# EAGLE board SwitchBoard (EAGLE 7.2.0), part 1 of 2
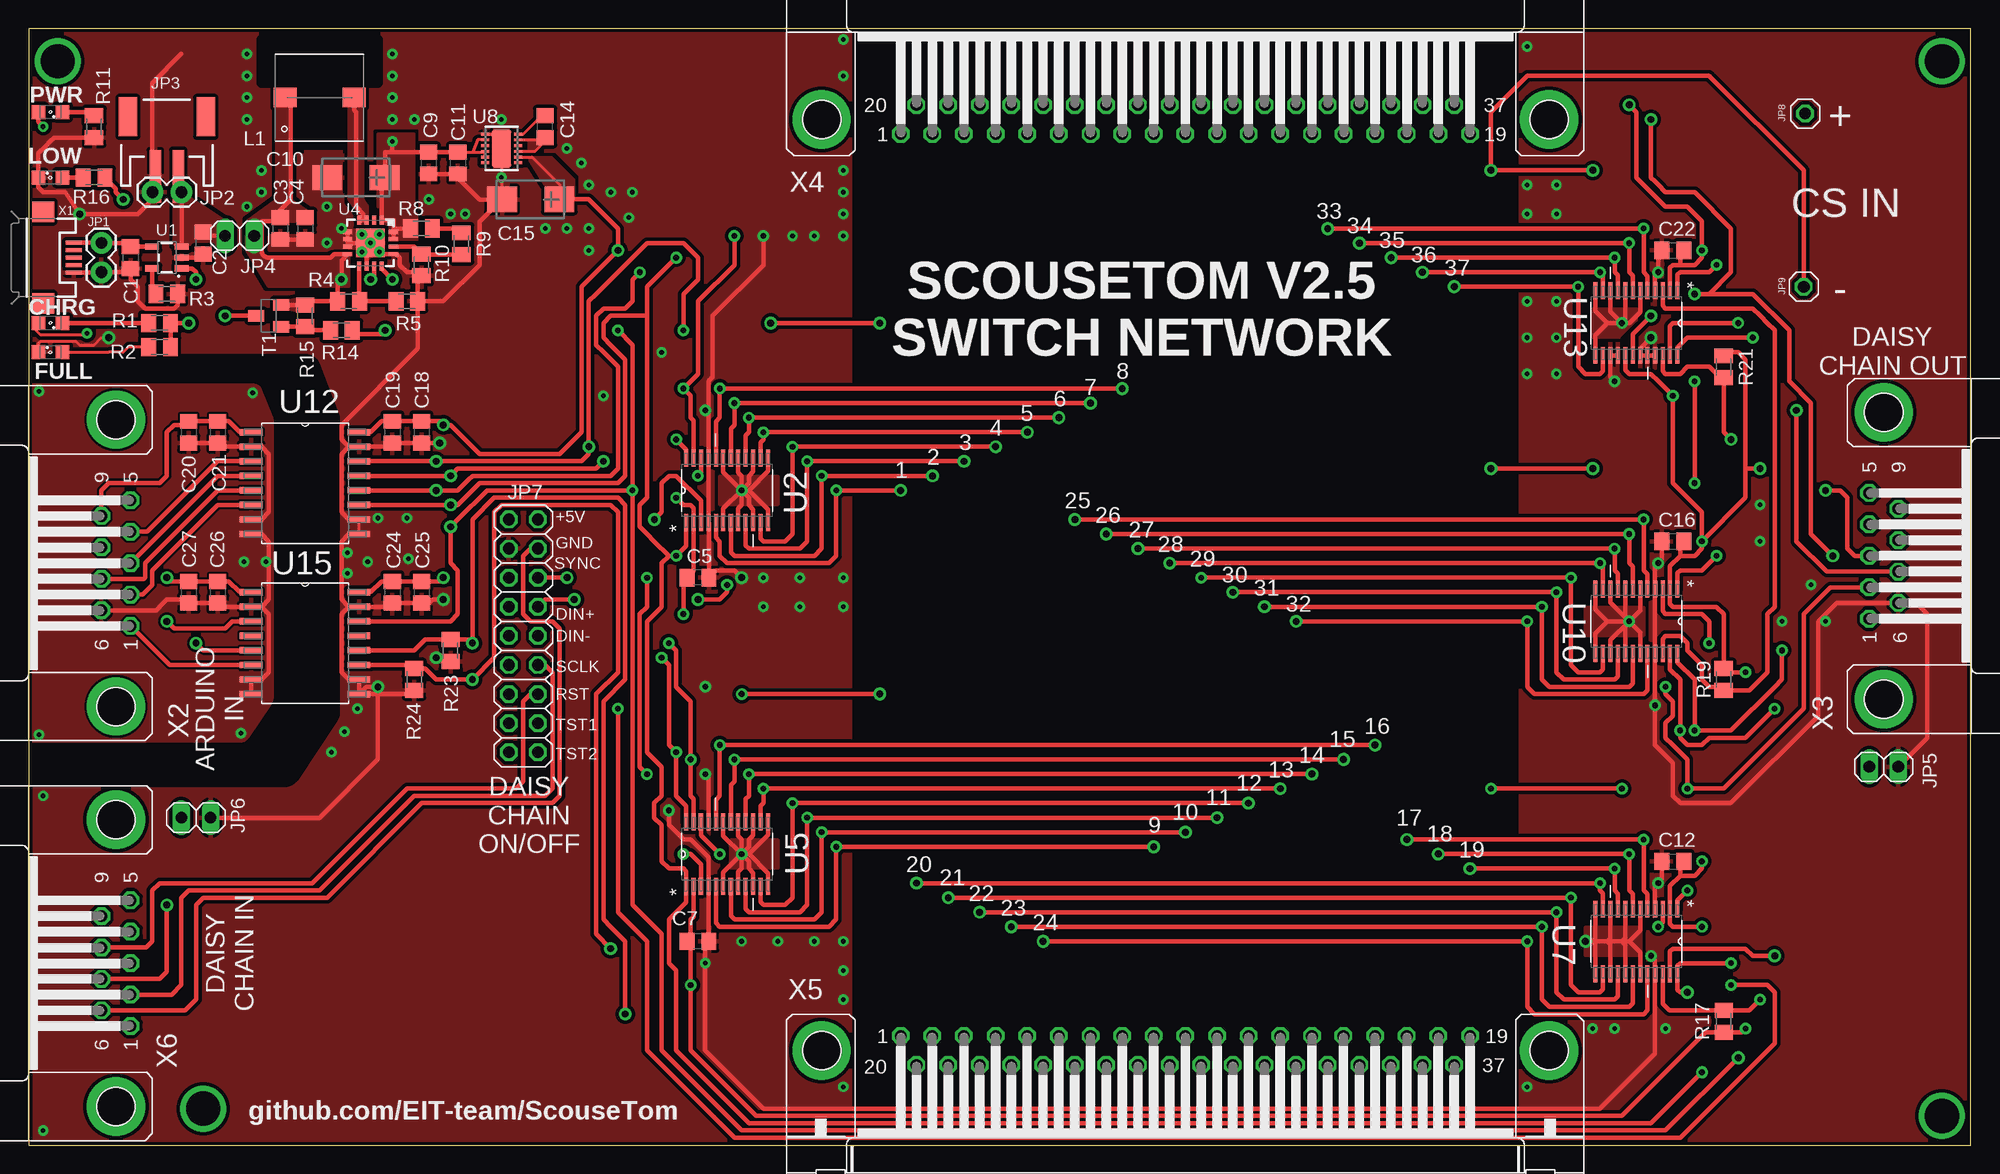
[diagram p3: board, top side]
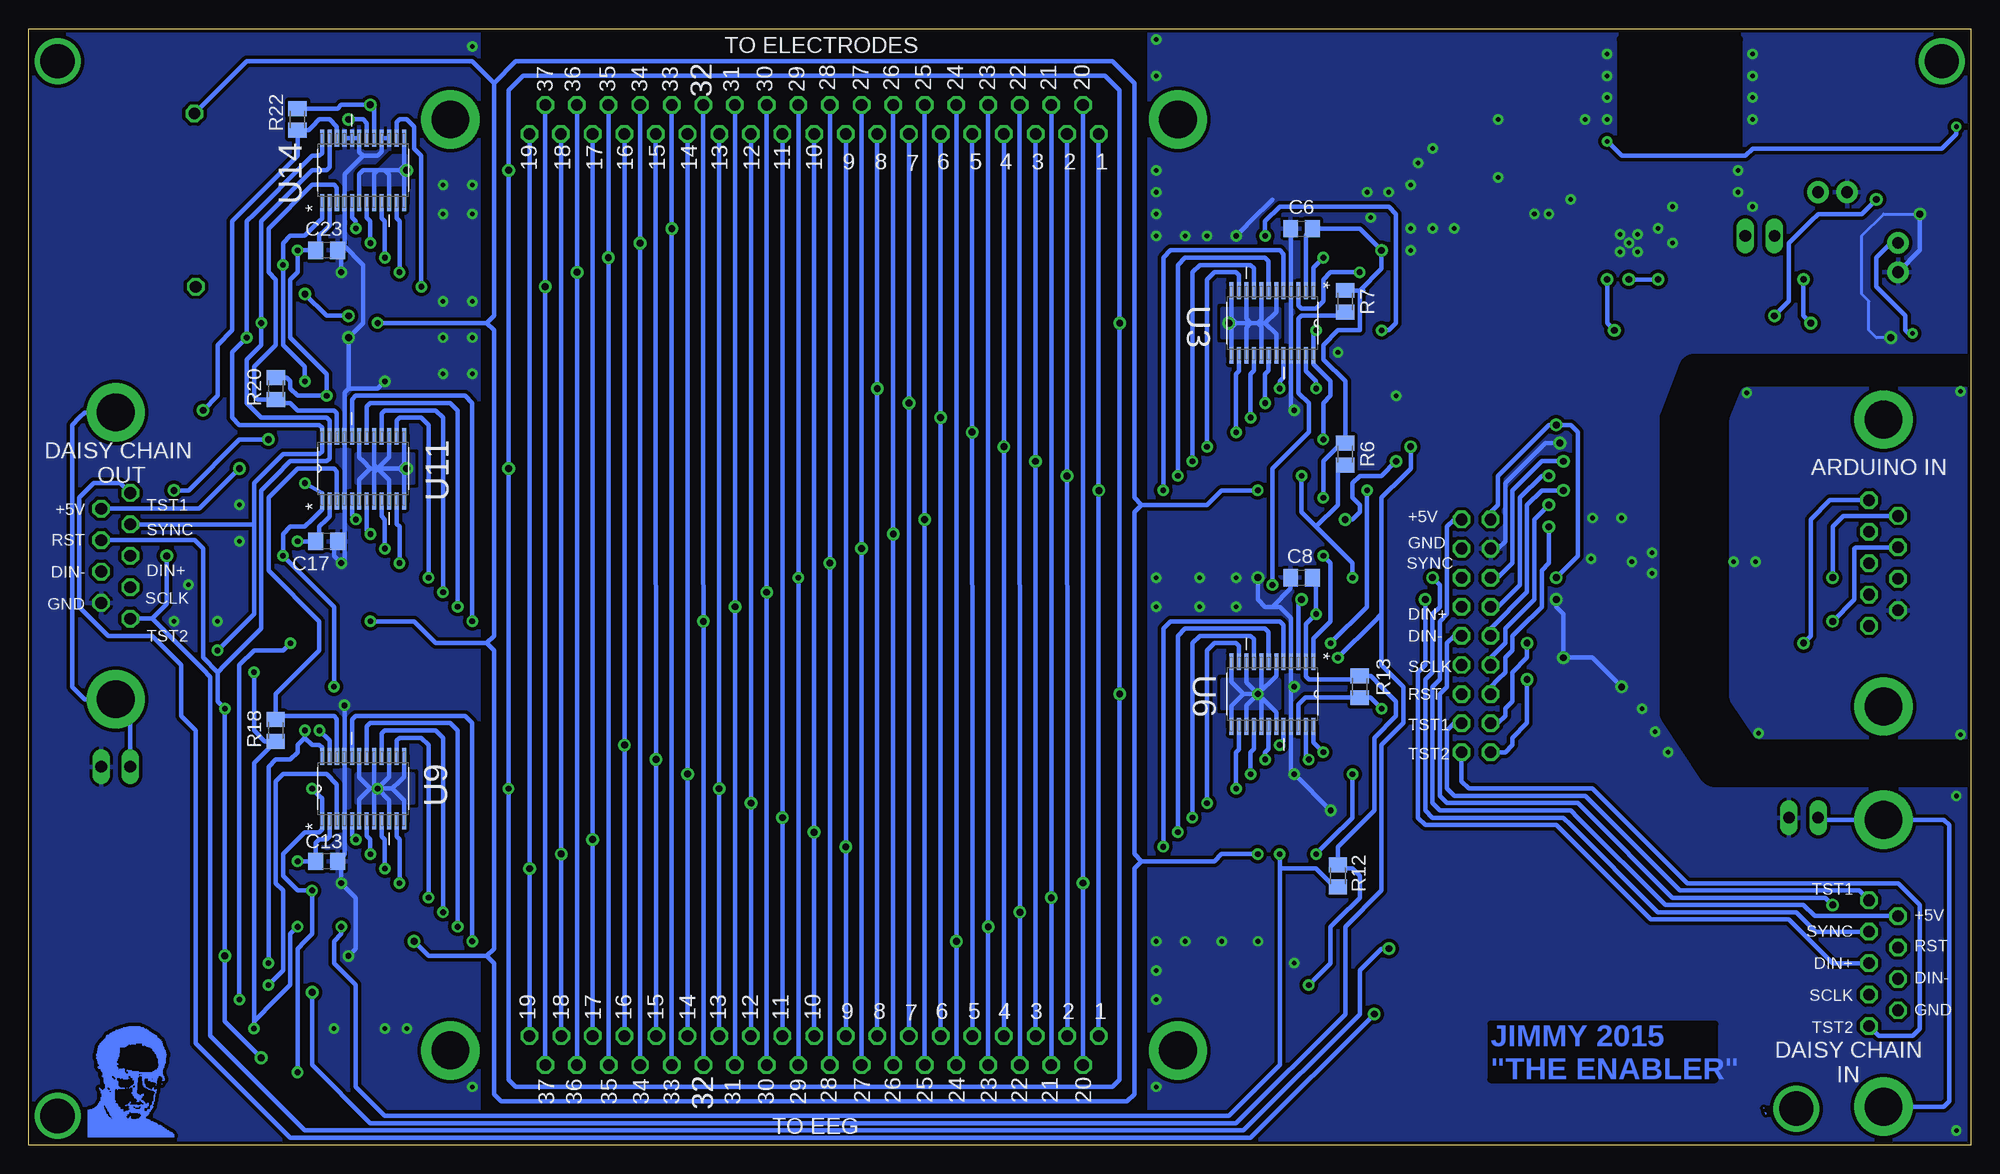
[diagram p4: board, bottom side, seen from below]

Size 169.53 x 97.46 mm. Coordinates in mm from the lower left corner, seen from the top.
Outline: 0,0 169.53,0 169.53,97.46 0,97.46 0,0
Copper layers (1*16): Top 0.035mm / dielectric 1.5mm / Bottom 0.035mm
Design rules "pcbtrain *": minimum track width 0.2mm, minimum drill 0.4mm, track to track 0.2mm, track to pad 0.2mm, pad to pad 0.2mm, via to via 0.2mm, smd to smd 0mil, copper to edge 10mil, drill to drill 0.2mm, minimum pad ring 10mil, minimum via ring 10mil, stop-mask expansion 0.125mm, vias tented up to drill 0mil, thermal gap 10mil
tRestrict: area 20.3,87 to 30.5,96.5; area -5.1,31.8 to 26.7,68.6; area 72.4,-1.3 to 129.5,100.3
bRestrict: area 20.3,87 to 30.5,96.5; area -5.1,31.8 to 26.7,68.6; area 72.4,-1.3 to 129.5,100.3

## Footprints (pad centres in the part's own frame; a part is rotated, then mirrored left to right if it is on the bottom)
C0805 = smd 1.3 x 1.5: 1 -0.95,0; 2 0.95,0
CT6032 = smd 2.6 x 2.2: + -2.5,0; - 2.5,0
1X02 = drill 1.016 pad 1.88: 1 0,0; 2 2.54,0
JST-2-SMD = smd 1 x 4.6: 1 -1,-3.7; 2 1,-3.7 | smd 1.6 x 3.4: NC1 -3.4,1.5; NC2 3.4,1.5
1X02' = drill 1.016 long: 1 -1.27,0; 2 1.27,0
2X09 = drill 1.016 octagon: 1 -10.16,-1.27; 2 -10.16,1.27; 3 -7.62,-1.27; 4 -7.62,1.27; 5 -5.08,-1.27; 6 -5.08,1.27; 7 -2.54,-1.27; 8 -2.54,1.27; 9 0,-1.27; 10 0,1.27; 11 2.54,-1.27; 12 2.54,1.27; 13 5.08,-1.27; 14 5.08,1.27; 15 7.62,-1.27; 16 7.62,1.27; 17 10.16,-1.27; 18 10.16,1.27
1X01 = drill 1.016 octagon: 1 0,0
WE-PD_7332/7345_PLASTIC_BASE = smd 1.7 x 2: 1 0,3; 2 0,-3
SML0805 = smd 1.2 x 1.2: A 1.05,0; C -1.05,0
M0805 = smd 1.3 x 1.6: 1 -0.95,0; 2 0.95,0
SOT23-BEC = smd 1 x 1.4: B -0.95,-1.1; C 0,1.1; E 0.95,-1.1
SOT23-5 = smd 0.55 x 1.2: 1 -0.95,-1.3; 2 0,-1.3; 3 0.95,-1.3; 4 0.95,1.3; 5 -0.95,1.3
SOP65P640X120-24N = smd 1.473 x 0.356: 1 -2.819,3.581; 2 -2.819,2.921; 3 -2.819,2.286; 4 -2.819,1.626; 5 -2.819,0.965; 6 -2.819,0.33; 7 -2.819,-0.33; 8 -2.819,-0.965; 9 -2.819,-1.626; 10 -2.819,-2.286; 11 -2.819,-2.921; 12 -2.819,-3.581; 13 2.819,-3.581; 14 2.819,-2.921; 15 2.819,-2.286; 16 2.819,-1.626; 17 2.819,-0.965; 18 2.819,-0.33; 19 2.819,0.33; 20 2.819,0.965; 21 2.819,1.626; 22 2.819,2.286; 23 2.819,2.921; 24 2.819,3.581
QFN16-4X4 = smd 0.8 x 0.35: 1 -2,0.975; 2 -2,0.325; 3 -2,-0.325; 4 -2,-0.975; 9 2,-0.975; 10 2,-0.325; 11 2,0.325; 12 2,0.975 | smd 0.35 x 0.8: 5 -0.975,-2; 6 -0.325,-2; 7 0.325,-2; 8 0.975,-2; 13 0.975,2; 14 0.325,2; 15 -0.325,2; 16 -0.975,2 | smd 2.5 x 2.5: EXP 0,0
DFN12 = smd 0.25 x 0.7: 1 -1.25,-1.45; 2 -0.75,-1.45; 3 -0.25,-1.45; 4 0.25,-1.45; 5 0.75,-1.45; 6 1.25,-1.45; 7 1.25,1.45; 8 0.75,1.45; 9 0.25,1.45; 10 -0.25,1.45; 11 -0.75,1.45; 12 -1.25,1.45 | smd 3.3 x 1.7: EXP 0,0
SOIC127P1032X265-16N = smd 1.981 x 0.559: 1 -4.699,4.445; 2 -4.699,3.175; 3 -4.699,1.905; 4 -4.699,0.635; 5 -4.699,-0.635; 6 -4.699,-1.905; 7 -4.699,-3.175; 8 -4.699,-4.445; 9 4.699,-4.445; 10 4.699,-3.175; 11 4.699,-1.905; 12 4.699,-0.635; 13 4.699,0.635; 14 4.699,1.905; 15 4.699,3.175; 16 4.699,4.445
USB-MICROB = smd 0.35 x 1.4: D+ 0,2.65; D- -0.65,2.65; GND 1.3,2.65; ID 0.65,2.65; VBUS -1.3,2.65 | smd 1.8 x 1.9: MT1 -4,0; MT2 4,0
F09HP = drill 1.016 octagon: 1 -5.486,-1.27; 2 -2.743,-1.27; 3 0,-1.27; 4 2.743,-1.27; 5 5.486,-1.27; 6 -4.115,1.27; 7 -1.372,1.27; 8 1.372,1.27; 9 4.115,1.27 | drill 3.302 pad 5.08: G1 -12.522,0; G2 12.522,0
M09HP = drill 1.016 octagon: 1 -5.486,1.27; 2 -2.743,1.27; 3 0,1.27; 4 2.743,1.27; 5 5.486,1.27; 6 -4.115,-1.27; 7 -1.372,-1.27; 8 1.372,-1.27; 9 4.115,-1.27 | drill 3.302 pad 5.08: G1 -12.522,0; G2 12.522,0
F37HP = drill 1.016 octagon: 1 -24.841,-1.27; 2 -22.073,-1.27; 3 -19.329,-1.27; 4 -16.561,-1.27; 5 -13.792,-1.27; 6 -11.049,-1.27; 7 -8.28,-1.27; 8 -5.512,-1.27; 9 -2.769,-1.27; 10 0,-1.27; 11 2.769,-1.27; 12 5.512,-1.27; 13 8.28,-1.27; 14 11.049,-1.27; 15 13.818,-1.27; 16 16.561,-1.27; 17 19.329,-1.27; 18 22.098,-1.27; 19 24.841,-1.27; 20 -23.47,1.27; 21 -20.701,1.27; 22 -17.932,1.27; 23 -15.189,1.27; 24 -12.421,1.27; 25 -9.652,1.27; 26 -6.909,1.27; 27 -4.14,1.27; 28 -1.372,1.27; 29 1.372,1.27; 30 4.14,1.27; 31 6.909,1.27; 32 9.677,1.27; 33 12.421,1.27; 34 15.189,1.27; 35 17.958,1.27; 36 20.701,1.27; 37 23.47,1.27 | drill 3.302 pad 5.08: G1 -31.75,0; G2 31.75,0
M37HP = drill 1.016 octagon: 1 -24.841,1.27; 2 -22.098,1.27; 3 -19.329,1.27; 4 -16.561,1.27; 5 -13.818,1.27; 6 -11.049,1.27; 7 -8.28,1.27; 8 -5.512,1.27; 9 -2.769,1.27; 10 0,1.27; 11 2.769,1.27; 12 5.512,1.27; 13 8.28,1.27; 14 11.049,1.27; 15 13.792,1.27; 16 16.561,1.27; 17 19.329,1.27; 18 22.073,1.27; 19 24.841,1.27; 20 -23.47,-1.27; 21 -20.701,-1.27; 22 -17.958,-1.27; 23 -15.189,-1.27; 24 -12.421,-1.27; 25 -9.652,-1.27; 26 -6.909,-1.27; 27 -4.14,-1.27; 28 -1.372,-1.27; 29 1.372,-1.27; 30 4.14,-1.27; 31 6.909,-1.27; 32 9.652,-1.27; 33 12.421,-1.27; 34 15.189,-1.27; 35 17.932,-1.27; 36 20.701,-1.27; 37 23.47,-1.27 | drill 3.302 pad 5.08: G1 -31.75,0; G2 31.75,0

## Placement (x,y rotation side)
C1  10uF  [C0805]  8.89,77.47 270 top
C2  10uF  [C0805]  15.24,78.74 270 top
C3  10uF  [C0805]  21.97,80.01 270 top
C4  0.1uF  [C0805]  24.13,80.01 270 top
C5  0.1uF  [C0805]  58.42,49.53 180 top
C6  0.1uF  [C0805]  58.42,80.01 0 bottom
C7  0.1uF  [C0805]  58.42,17.78 180 top
C8  0.1uF  [C0805]  58.42,49.53 0 bottom
C9  2.2uF  [C0805]  34.92,85.72 270 top
C10  100uF  [CT6032]  28.57,84.46 180 top
C11  10uF  [C0805]  37.47,85.72 270 top
C12  0.1uF  [C0805]  143.51,24.76 0 top
C13  0.1uF  [C0805]  143.51,24.77 180 bottom
C14  0.01uF  [C0805]  45.09,88.9 90 top
C15  100uF  [CT6032]  43.81,82.55 180 top
C16  0.1uF  [C0805]  143.51,52.7 0 top
C17  0.1uF  [C0805]  143.51,52.71 180 bottom
C18  .1uF  [C0805]  34.29,62.23 270 top
C19  1uF  [C0805]  31.75,62.23 270 top
C20  .1uF  [C0805]  13.97,62.23 270 top
C21  1uF  [C0805]  16.51,62.23 270 top
C22  0.1uF  [C0805]  143.51,78.1 0 top
C23  0.1uF  [C0805]  143.51,78.11 180 bottom
C24  .1uF  [C0805]  31.75,48.26 270 top
C25  1uF  [C0805]  34.29,48.26 270 top
C26  .1uF  [C0805]  16.51,48.26 270 top
C27  1uF  [C0805]  13.97,48.26 270 top
JP1  IN  [1X02]  6.35,78.74 270 top
JP2  LiPoIN  [1X02]  13.34,83.18 180 top
JP3  LiPo  [JST-2-SMD]  12.07,88.26 0 top
JP4  PWR  [1X02']  18.41,79.38 0 top
JP5  Shld  [1X02']  161.93,33.02 180 top
JP6  Shld  [1X02']  14.61,28.57 0 top
JP7  DCHN  [2X09]  43.18,44.45 270 top
JP8  CS_IN+  [1X01]  155.07,90.04 0 top
JP9  CS_IN-  [1X01]  154.94,74.93 0 top
L1  6.8uH  [WE-PD_7332/7345_PLASTIC_BASE]  25.4,91.44 90 top
LED1  YELLOW  [SML0805]  1.9,71.75 180 top
LED2  GREEN  [SML0805]  1.9,69.22 0 top
LED3  GREEN  [SML0805]  1.9,90.17 180 top
LED4  RED  [SML0805]  1.9,84.46 0 top
R1  470  [M0805]  11.43,71.75 180 top
R2  1k  [M0805]  11.43,69.66 180 top
R3  2k  [M0805]  12.06,74.29 180 top
R4  2M  [M0805]  27.94,73.66 180 top
R5  360k  [M0805]  33.02,73.66 180 top
R6  10k  [M0805]  54.61,60.33 90 bottom
R7  10k  [M0805]  54.61,73.66 90 bottom
R8  1.8M  [M0805]  34.29,80.01 180 top
R9  82k  [M0805]  37.78,78.68 90 top
R10  200k  [M0805]  34.29,76.84 90 top
R11  1k  [M0805]  5.71,88.9 270 top
R12  10k  [M0805]  55.25,23.5 90 bottom
R13  10k  [M0805]  53.34,40 90 bottom
R14  4.7k  [M0805]  27.3,71.12 180 top
R15  47k  [M0805]  24.13,72.39 90 top
R16  1k  [M0805]  5.71,84.46 180 top
R17  10k  [M0805]  147.96,10.8 270 top
R18  10k  [M0805]  147.96,36.2 270 bottom
R19  10k  [M0805]  147.95,40.64 90 top
R20  10k  [M0805]  147.95,66.04 90 bottom
R21  10k  [M0805]  147.96,67.94 90 top
R22  10k  [M0805]  146.05,89.53 90 bottom
R23  10M  [M0805]  36.83,43.18 90 top
R24  10M  [M0805]  33.66,40.64 90 top
T1  PNP  [SOT23-BEC]  20.95,72.39 90 top
U1  MCP73831  [SOT23-5]  12.06,77.47 90 top
U2  ADG714BRUZ  [SOP65P640X120-24N]  60.96,57.15 90 top
U3  ADG714BRUZ  [SOP65P640X120-24N]  60.96,71.76 270 bottom
U4  TPS61090RSAR  [QFN16-4X4]  29.84,78.74 270 top
U5  ADG714BRUZ  [SOP65P640X120-24N]  60.96,25.4 90 top
U6  ADG714BRUZ  [SOP65P640X120-24N]  60.96,39.37 270 bottom
U7  ADG714BRUZ  [SOP65P640X120-24N]  140.34,17.78 270 top
U8  LT1763CDE-5  [DFN12]  41.27,87 90 top
U9  ADG714BRUZ  [SOP65P640X120-24N]  140.33,31.12 90 bottom
U10  ADG714BRUZ  [SOP65P640X120-24N]  140.34,45.72 270 top
U11  ADG714BRUZ  [SOP65P640X120-24N]  140.33,59.06 90 bottom
U12  ADUM1410ARWZ  [SOIC127P1032X265-16N]  24.13,57.78 0 top
U13  ADG714BRUZ  [SOP65P640X120-24N]  140.34,71.75 270 top
U14  ADG714BRUZ  [SOP65P640X120-24N]  140.33,85.09 90 bottom
U15  ADUM1412ARWZ  [SOIC127P1032X265-16N]  24.13,43.81 0 top
X1  USB-MICROB  [USB-MICROB]  1.27,77.47 270 top
X2  CTR_ARD  [F09HP]  7.62,50.8 90 top
X3  CTR_OUT  [M09HP]  161.93,51.44 90 top
X4  DSUB _T  [F37HP]  100.96,89.54 0 top
X5  DSUB_B  [M37HP]  100.96,8.25 0 top
X6  CTR_IN  [F09HP]  7.62,15.88 90 top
